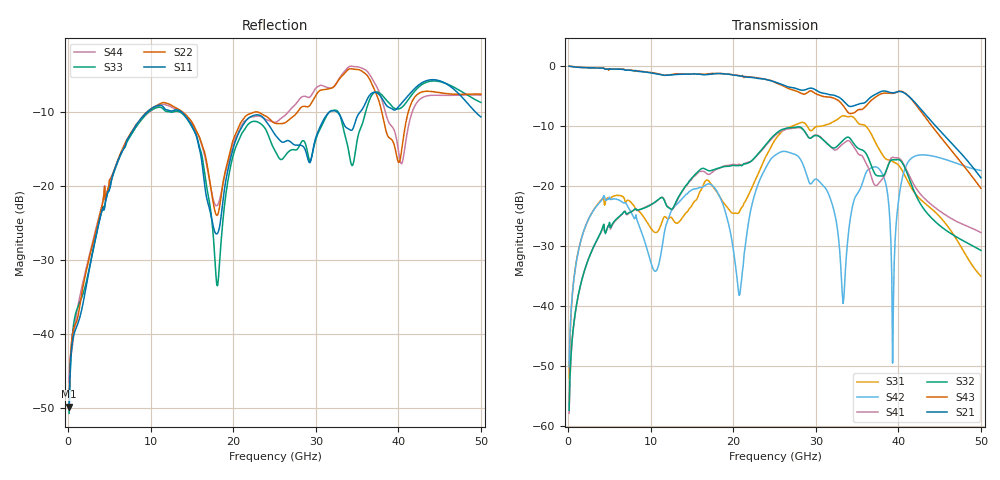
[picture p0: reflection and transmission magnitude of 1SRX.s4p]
! DAC39RF10ACK
! 256-pin FCBGA package
! Texas Instruments 8/20/2022
! Single-ended  S-parameters
! PORT#  PORT_NAME  NET_NAME
! PORT1:  xSRXN.DIEBUMP  xSRXN
! PORT2:  xSRXN.BGA  xSRXN
! PORT3:  xSRXP.DIEBUMP  xSRXP
! PORT4:  xSRXP.BGA  xSRXP
! Touchstone Ver. 1.0
! Number of ports is 4
# Hz	S	MA	R	50.000000
! SCATTERING PARAMETERS  :
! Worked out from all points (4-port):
!   500 points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, 100 MHz to 50 GHz, reference 50 ohm
!   strongest paths, dB at 100 MHz, 12.6 GHz, 25.1 GHz, 37.6 GHz, 50 GHz:
!     S21: 0.0, -1.5, -2.7, -4.4, -18.6
!     S43: 0.0, -1.4, -2.8, -4.9, -20.4
!     S32: -57.4, -23.8, -11.4, -18.3, -30.8
!     S41: -57.9, -23.9, -11.5, -19.6, -27.8
!     S42: -50.2, -23.9, -14.9, -17.1, -17.4
!     S31: -52.1, -25.4, -12.2, -13.7, -35.1
!   lowest |S11| = -49.9 dB at 100 MHz (marker M1), VSWR 1.01, Z = 50.3 + j0.134 ohm
!   |S11| at or under -10 dB: start of sweep to 9.542 GHz; 13.75 GHz to 31.61 GHz (17.86 GHz wide, 78.8 % of centre); 32.6 GHz to 35.35 GHz (2.752 GHz wide, 8.1 % of centre)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
1e8  0.003206 24.5  0.9955 -2.0  0.002536 85.5  0.001502 -103.9
     0.9965 -1.9  0.003559 25.8  0.001141 -97.3  0.003045 81.0
     0.002492 86.3  0.001342 -101.0  0.002891 23.8  0.9946 -2.1
     0.001266 -99.9  0.003107 81.1  0.9972 -1.8  0.004692 27.1
4.2e9  0.07101 27.5  0.9559 -73.2  0.07951 6.7  0.0459 -174.4
       0.9603 -73.1  0.07856 -16.4  0.04603 -173.2  0.07941 19.9
       0.07892 7.1  0.04599 -173.8  0.07303 31.9  0.9566 -72.6
       0.04526 -174.3  0.07947 19.8  0.9663 -72.2  0.0794 -17.6
1.01e10  0.3354 -71.7  0.876 -172.9  0.04453 -124.7  0.07026 84.4
         0.8744 -173.0  0.335 -98.1  0.07022 86.5  0.02176 -119.3
         0.04344 -124.9  0.07007 86.5  0.3277 -69.3  0.8765 -171.3
         0.07033 83.7  0.0219 -120.1  0.8817 -171.4  0.3248 -97.6
1.81e10  0.04795 -100.9  0.8637 55.2  0.08709 -68.0  0.1388 -43.0
         0.8654 55.2  0.06385 -124.3  0.1409 -42.5  0.08822 -2.3
         0.08681 -67.6  0.14 -42.5  0.02113 -106.4  0.8671 56.7
         0.1387 -43.2  0.08785 -2.2  0.8677 56.8  0.07438 -124.7
2.06e10  0.2257 -76.2  0.8285 9.7  0.05995 178.2  0.15 -89.4
         0.8292 9.7  0.2467 -97.4  0.147 -85.8  0.01377 14.3
         0.05915 177.8  0.1476 -85.5  0.2007 -72.5  0.8332 11.6
         0.1513 -88.7  0.01362 10.5  0.8359 11.4  0.2291 -96.8
3.03e10  0.2358 -89.2  0.6167 -157.6  0.3154 -136.7  0.2639 63.7
         0.6128 -157.8  0.4338 -121.7  0.2616 69.4  0.1097 -141.7
         0.3136 -137.6  0.2604 69.6  0.2297 -87.6  0.5713 -154.9
         0.263 63.7  0.1111 -142.4  0.5753 -154.4  0.473 -126.2
5e10  0.2936 -149.1  0.1098 -132.1  0.02781 4.7  0.03287 101.5
      0.117 -137.3  0.4194 -162.7  0.0369 117.7  0.1333 18.8
      0.01764 -17.5  0.02898 114.5  0.3682 -144.9  0.08736 -122.9
      0.04078 97.8  0.1343 19.5  0.09562 -122.6  0.4122 -163.9
